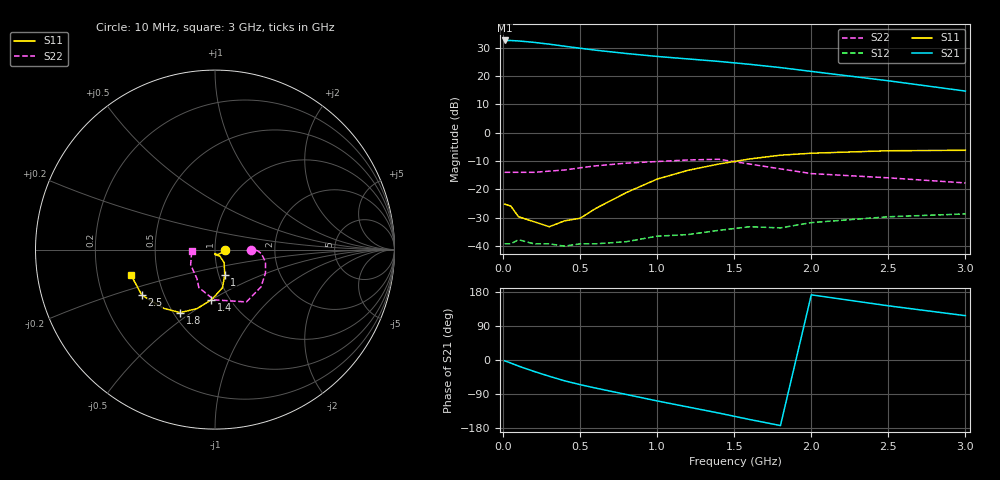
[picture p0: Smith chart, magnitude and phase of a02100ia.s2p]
!  INA-02100  S PARAMETERS
!  Id = 35 mA  LAST UPDATED 06-23-94
# ghz s ma r 50
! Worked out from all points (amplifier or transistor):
!   17 points, 10 MHz to 3 GHz, reference 50 ohm
!   highest |S21| = 32.5 dB at 10 MHz (marker M1)
!   |S21| within 3 dB of that: start of sweep to 538 MHz
!   unconditionally stable (mu >= 1): start of sweep to end of sweep
!   at 100 MHz: K = 1.16, MAG = 32.6 dB, |S12| = -37.7 dB
!   at 800 MHz: K = 1.65, MAG = 28.4 dB, |S12| = -38.4 dB
!   at 3 GHz: K = 1.93, MAG = 16.1 dB, |S12| = -28.6 dB
!   S11 on the Smith chart (normalised r, x): 10 MHz: 1.12, -0.01; 1 GHz: 1.07, -0.31; 1.4 GHz: 0.82, -0.50; 1.8 GHz: 0.54, -0.45; 2.5 GHz: 0.38, -0.25; 3 GHz: 0.35, -0.13
0.01  0.055 -4.0  42.1 -2.0  0.011 14.0  0.2 0.0
0.05  0.051 -11.0  42 -8.0  0.011 12.0  0.2 -1.0
0.1  0.033 -56.0  41.3 -16.0  0.013 6.0  0.2 -2.0
0.2  0.027 -75.0  39 -30.0  0.011 -4.0  0.2 0.0
0.3  0.022 -93.0  36.2 -43.0  0.011 -13.0  0.21 1.0
0.4  0.028 -89.0  33.3 -55.0  0.01 -3.0  0.22 0.0
0.5  0.031 -77.0  30.7 -65.0  0.011 -19.0  0.24 -2.0
0.6  0.046 -53.0  28.4 -74.0  0.011 -7.0  0.26 -5.0
0.8  0.088 -55.0  24.8 -91.0  0.012 -12.0  0.29 -14.0
1  0.152 -69.0  22 -108.0  0.015 -21.0  0.31 -25.0
1.2  0.217 -79.0  19.9 -124.0  0.016 -19.0  0.33 -39.0
1.4  0.28 -94.0  18 -140.0  0.019 -18.0  0.34 -59.0
1.6  0.344 -107.0  16 -157.0  0.022 -31.0  0.28 -91.0
1.8  0.401 -119.0  14 -173.0  0.021 -27.0  0.23 -113.0
2  0.434 -131.0  12 172.0  0.026 -29.0  0.19 -122.0
2.5  0.48 -148.0  8.2 143.0  0.033 -41.0  0.16 -148.0
3  0.489 -163.0  5.4 117.0  0.037 -42.0  0.13 -176.0
